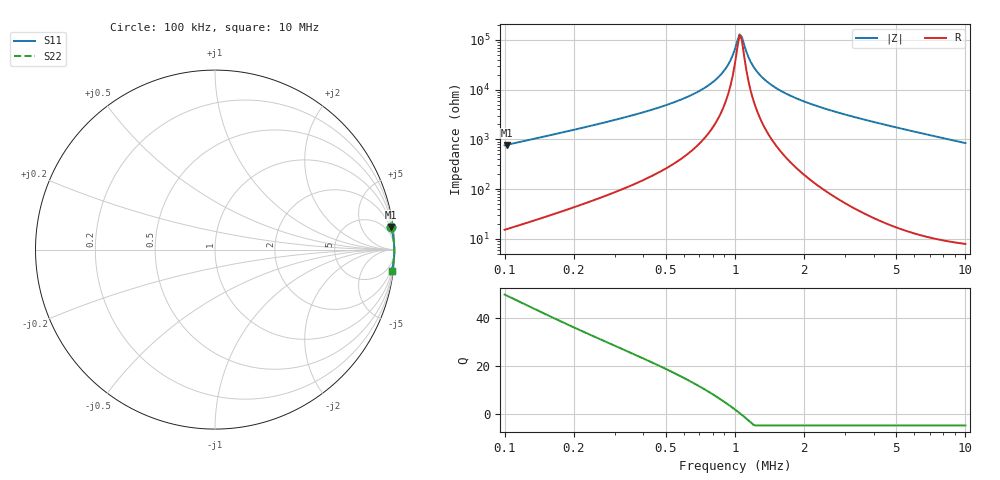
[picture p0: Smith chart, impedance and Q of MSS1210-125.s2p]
# MHz S MA R 50
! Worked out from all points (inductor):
!   203 points, 100 kHz to 10 MHz, reference 50 ohm
!   read as one part in series: L = 1.2 mH near 102.3 kHz
!   highest Q = 49.5 at 102.3 kHz (marker M1), where L = 1.21 mH
!   self-resonance near 1.047 MHz
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0.1  0.9889 7.5  0.13 -81.4  0.13 -81.4  0.9889 7.5
0.102306  0.9893 7.3  0.1271 -81.5  0.1271 -81.5  0.9893 7.3
0.1728318  0.9953 4.3  0.07435 -84.3  0.07435 -84.3  0.9953 4.3
0.2726739  0.9975 2.6  0.04529 -85.5  0.04529 -85.5  0.9975 2.6
0.6943591  0.999 0.6  0.01082 -84.5  0.01082 -84.5  0.999 0.6
0.8524974  0.9991 0.3  0.00542 -80.8  0.00542 -80.8  0.9991 0.3
0.9128429  0.9992 0.2  0.003696 -77.1  0.003696 -77.1  0.9992 0.2
0.9554281  0.9992 0.1  0.002575 -71.9  0.002575 -71.9  0.9992 0.1
1  0.9992 0.1  0.001512 -59.0  0.001512 -59.0  0.9992 0.1
1.046651  0.9992 0.0  0.0007741 -11.1  0.0007741 -11.1  0.9992 0.0
1.070787  0.9992 -0.0  0.0008632 29.5  0.0008632 29.5  0.9992 -0.0
1.12074  0.9993 -0.1  0.001737 64.9  0.001737 64.9  0.9993 -0.1
1.173024  0.9993 -0.2  0.00282 75.1  0.00282 75.1  0.9993 -0.2
1.285023  0.9993 -0.3  0.005098 81.9  0.005098 81.9  0.9993 -0.3
1.473387  0.9993 -0.5  0.008647 85.2  0.008647 85.2  0.9993 -0.5
1.768173  0.9993 -0.8  0.01366 86.7  0.01366 86.7  0.9993 -0.8
2.43298  0.9992 -1.4  0.02365 87.3  0.02365 87.3  0.9992 -1.4
3.424944  0.9988 -2.1  0.03707 87.1  0.03707 87.1  0.9988 -2.1
5.162633  0.9977 -3.4  0.05908 86.1  0.05908 86.1  0.9977 -3.4
6.787083  0.9962 -4.5  0.07897 85.0  0.07897 85.0  0.9962 -4.5
8.524974  0.9941 -5.7  0.09988 83.8  0.09988 83.8  0.9941 -5.7
10  0.992 -6.7  0.1174 82.7  0.1174 82.7  0.992 -6.7
